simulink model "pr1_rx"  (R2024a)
settings: Solver=FixedStepDiscrete  StartTime=0.0  StopTime=0.5  RelTol=1e-3
undefined symbols (not defined in the file or in its folder): Fs, ip
libraries: ad936xlib x1

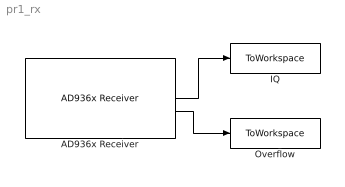
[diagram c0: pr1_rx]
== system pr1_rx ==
  AD936x Receiver : ad936xlib/AD936x Receiver  IPAddress=169.254.0.52  uri=ip:10.0.0.200  CenterFrequencySource=Dialog  CenterFrequency=c.RF  GainSource=AGC Slow Attack  GainSourceBlock=Dialog  Gain=30  ChannelMapping=1  BasebandSampleRate=c.Fs  OutputDataType=double  SamplesPerFrame=c.CaptureLength  OverflowOutputPort=on  EnableBurstMode=off  NumFramesInBurst=1  ShowAdvancedProperties=off  UseCustomFilter=off  filtPathRates=[737280000 11520000 3840000 1920000 960000 240000]  filtCoefficients="[-192 82 85 -215 228 -102 -110 290 -318 145 160 -426 471 -215 -238 633 -697 318 349 -923 1009 -457 -498 1309 -1423 640 693 -1812 1959 -876 -945 2458 -2647 1180 1268 -3290 3534 -1572 -1688 4375 -4698 2091 2247 -5836 6284 -2807 -3031 7918 -8588 3870 4225 -11182 12324 -5662 -6330 17255 -19735 9507 11312 -33568 43355 -25227 -42139 305542 305542 -42139 -25227 43355 -33568 11312 9507 -19735 17255 -6330 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"  filtCoefficientSize=128  filtDecimInterpFactor=4  filtGain=-12  filtRFBandwidth=18000000  filterConfigStruct=struct()  BypassUserLogic=off  EnableQuadratureCorrection=on  EnableRFDCCorrection=on  EnableBasebandDCCorrection=on  OverrideSampleTime=off  SampleTime=0.02  DataTimeout=Inf  ENSMPinControlMode=None  BISTLoopbackMode=Disabled  BISTToneInject=Disabled  BISTSignalGen=PRBS  BISTToneFreq=Fs/32  BISTToneLevel=0
  IQ : ToWorkspace  VariableName=rxIQ  SampleTime=-1
  Overflow : ToWorkspace  VariableName=rxOverflow  SampleTime=-1
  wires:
  AD936x Receiver/2 -> Overflow/1
  AD936x Receiver/1 -> IQ/1
